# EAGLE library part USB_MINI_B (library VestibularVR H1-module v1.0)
CONN RCPT USB2.0 MINI B SMD R/A
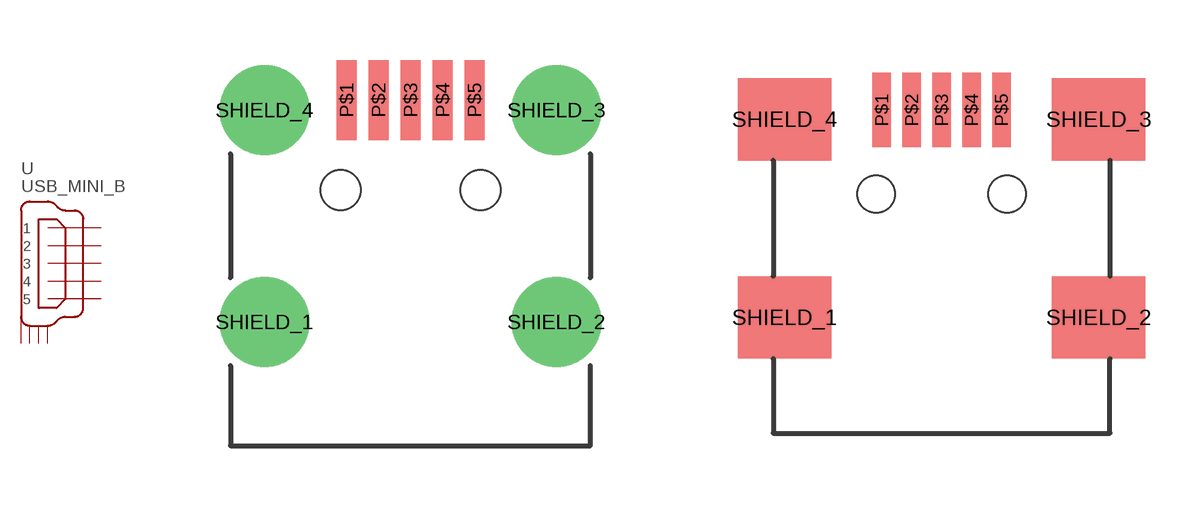
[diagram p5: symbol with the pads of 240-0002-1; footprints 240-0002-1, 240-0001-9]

Designator prefix -

## USB_MINI_B  [240-0002-1]
P$1  1
P$2  2
P$3  3
P$4  4
P$5  5
SHIELD_1  P$1
SHIELD_2  P$2
SHIELD_3  P$3
SHIELD_4  P$4

## USB_MINI_B""  [240-0001-9]
Pads as for 240-0002-1

## Footprint 240-0002-1 (pad centres in mm)
smd 0.5 x 2: P$1 -1.6,8.65; P$2 -0.8,8.65; P$3 0,8.65; P$4 0.8,8.65; P$5 1.6,8.65
drill 1.5: SHIELD_1 -3.65,3.1; SHIELD_2 3.65,3.1; SHIELD_3 3.65,8.4; SHIELD_4 -3.65,8.4
hole 1 at -1.75,6.4
hole 1 at 1.75,6.4

## Footprint 240-0001-9 (pad centres in mm)
smd 0.5 x 2: P$1 -1.6,8.65; P$2 -0.8,8.65; P$3 0,8.65; P$4 0.8,8.65; P$5 1.6,8.65
smd 2.5 x 2.2: SHIELD_1 -4.2,3.1; SHIELD_2 4.2,3.1; SHIELD_3 4.2,8.4; SHIELD_4 -4.2,8.4
hole 1 at -1.75,6.4
hole 1 at 1.75,6.4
